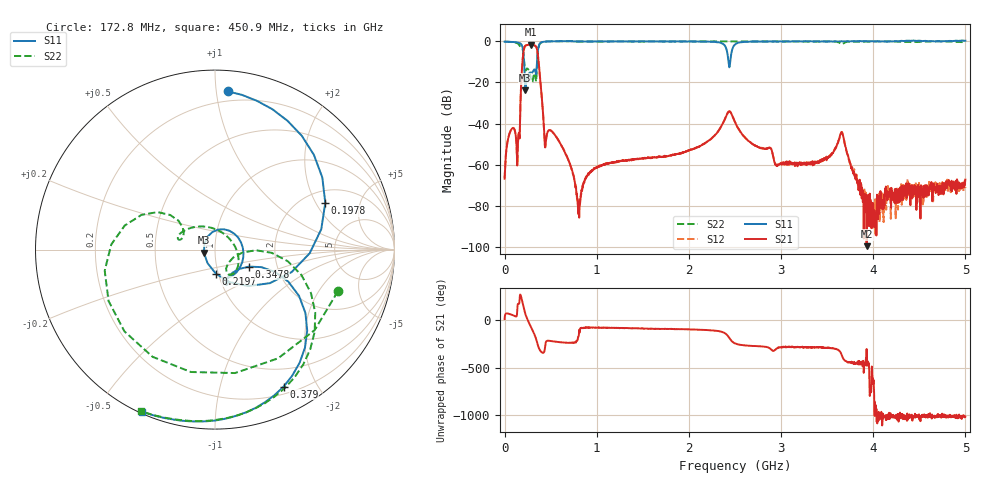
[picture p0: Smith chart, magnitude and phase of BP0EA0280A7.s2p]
!Agilent Technologies,E8358A,US41080443,A.07.50.56
!Agilent E8358A: A.07.50.56
!Date: Friday, November 10, 2017 09:06:09
!Correction: S11(Full 2 Port(1,2))
!S21(Full 2 Port(1,2))
!S12(Full 2 Port(1,2))
!S22(Full 2 Port(1,2))
!S2P File: Measurements: S11, S21, S12, S22:
# Hz S  dB  R 50
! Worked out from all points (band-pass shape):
!   1601 points, 1 MHz to 5 GHz, reference 50 ohm
!   highest |S21| = -1.61 dB at 282.2 MHz (marker M1); lowest = -99.6 dB at 3.928 GHz (marker M2)
!   |S21| within 3 dB of the highest: 207.6 MHz to 355.6 MHz (148 MHz wide, 52.6 % of centre)
!   lowest |S11| = -23.8 dB at 226 MHz (marker M3), VSWR 1.14, Z = 44.1 - j1.51 ohm
!   |S11| at or under -10 dB: 211.8 MHz to 352.6 MHz (140.8 MHz wide, 49.9 % of centre); 2.43 GHz to 2.448 GHz (18.43 MHz wide, 0.755 % of centre)
!   |S22| runs from -20.0 to 0.1 dB; largest |S21 - S12| = 0.0055
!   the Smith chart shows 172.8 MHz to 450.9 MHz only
!   S11 on the Smith chart (normalised r, x): 172.8 MHz: 0.13, +1.07; 197.8 MHz: 2.57, +2.40; 219.7 MHz: 0.97, -0.27; 347.8 MHz: 1.43, -0.28; 379 MHz: 0.28, -1.58; 450.9 MHz: 0.01, -0.65
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1000000  -0.17 179.7  -66.80 12.2  -66.49 12.8  -0.17 179.7
6.34875e7  -0.26 160.3  -43.77 63.1  -43.68 63.6  -0.29 157.3
1.322238e8  -0.52 127.6  -52.77 45.4  -52.83 46.0  -0.79 108.5
1.728406e8  -1.07 85.5  -30.47 -91.2  -30.43 -91.2  -2.82 -18.8
1.978356e8  -3.52 22.9  -8.43 178.3  -8.37 178.3  -4.07 -169.2
2.197062e8  -17.45 -88.0  -2.54 87.9  -2.49 87.9  -13.15 145.2
2.25955e8  -23.83 -164.6  -2.15 66.9  -2.10 67.0  -14.35 157.5
2.821938e8  -15.16 -56.8  -1.61 -61.8  -1.56 -61.7  -16.80 116.9
3.478056e8  -13.51 -26.6  -3.15 145.4  -3.10 145.5  -16.19 -5.9
3.790494e8  -1.38 -63.4  -14.36 52.0  -14.31 52.1  -1.53 -58.1
4.5091e8  -0.09 -114.1  -47.77 133.2  -47.71 133.3  -0.09 -114.5
8.352081e8  -0.05 -158.7  -72.17 -80.1  -73.25 -87.4  -0.08 -159.1
1.669416e9  -0.06 -177.7  -56.17 -91.7  -56.25 -93.3  -0.07 -177.8
2.391147e9  -2.13 126.1  -37.74 -136.9  -37.75 -136.7  -0.07 171.7
2.441137e9  -12.52 -18.1  -34.05 169.7  -34.06 169.8  -0.10 170.5
2.5005e9  -1.56 -142.2  -39.34 115.3  -39.34 115.3  -0.09 169.4
2.953534e9  -0.14 175.3  -60.07 61.3  -60.27 63.5  -0.08 163.4
3.334708e9  0.00 168.4  -58.68 73.2  -59.13 80.3  -0.06 158.3
3.659643e9  0.01 163.0  -44.30 -12.9  -44.35 -11.8  -1.45 156.5
3.928339e9  0.05 159.9  -99.62 56.5  -81.46 -49.7  -0.11 155.0
4.168916e9  0.03 157.4  -73.90 66.0  -73.80 61.4  -0.02 155.1
5e9  0.32 151.1  -67.20 63.5  -71.30 56.3  -0.45 156.3
